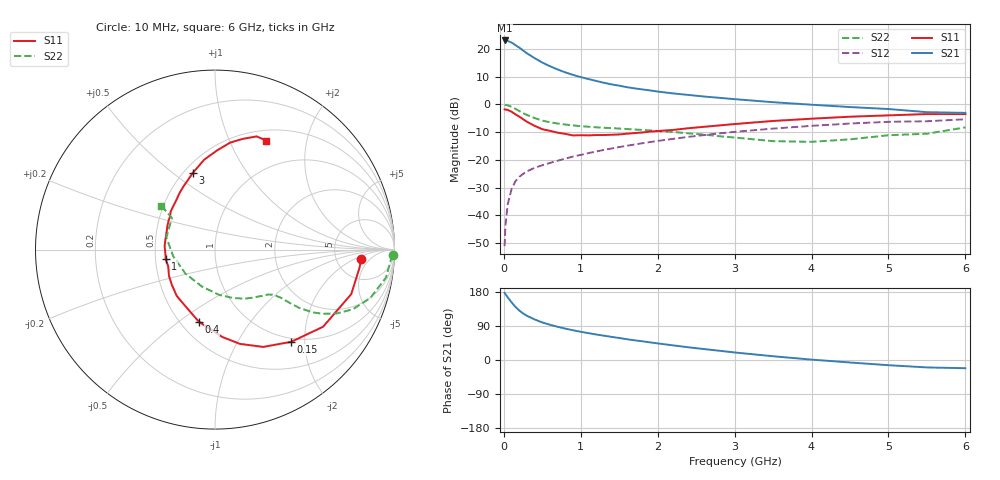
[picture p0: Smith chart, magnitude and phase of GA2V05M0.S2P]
! Infineon Technologies  Discrete & RF Semiconductors
! BF775
! Si NPN RF Bipolar Junction Transistor in SOT23
! VCE = 2 V  IC = 5 mA
! Common Emitter S-Parameters:  May  1996
# GHz  S  MA  R  50
!  f  S11  S21  S12  S22
! GHz  MAG  ANG  MAG  ANG  MAG  ANG  MAG  ANG
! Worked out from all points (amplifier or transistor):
!   36 points, 10 MHz to 6 GHz, reference 50 ohm
!   highest |S21| = 23.1 dB at 10 MHz (marker M1)
!   |S21| within 3 dB of that: start of sweep to 221 MHz
!   unconditionally stable (mu >= 1): 767.1 MHz to 3.983 GHz; 5.355 GHz to 5.765 GHz
!   at 250 MHz: K = 0.50, MSG = 22.2 dB, |S12| = -25.0 dB
!   at 1.4 GHz: K = 1.14, MAG = 9.2 dB, |S12| = -15.9 dB
!   at 6 GHz: K = 0.99, MSG = 1.2 dB, |S12| = -5.3 dB
!   lowest NFmin = 1.50 dB at 450 MHz
!   S11 on the Smith chart (normalised r, x): 10 MHz: 8.95, -2.91; 150 MHz: 0.93, -1.73; 400 MHz: 0.62, -0.60; 1 GHz: 0.57, -0.06; 3 GHz: 0.56, +0.59; 6 GHz: 0.63, +1.38
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0.01  0.8167 -3.8  14.24 177.2  0.0028 87.8  0.99 -1.8
0.02  0.8112 -7.3  14.04 173.9  0.0064 83.1  0.9798 -3.7
0.05  0.7986 -18.1  13.96 165.5  0.0158 79.7  0.966 -9.2
0.1  0.7399 -35.5  13.07 152.3  0.0296 71.6  0.9065 -17.3
0.15  0.6666 -50.4  11.74 140.3  0.0412 65.6  0.837 -23.4
0.2  0.6053 -63.6  10.61 130.7  0.0495 61.2  0.7639 -27.8
0.25  0.5433 -75.2  9.392 122.9  0.0561 57.9  0.6978 -30.8
0.3  0.4885 -85.2  8.358 116.7  0.0625 56.5  0.6474 -32.7
0.4  0.4118 -102.6  6.846 107.1  0.0721 54.1  0.5697 -34.7
0.5  0.3584 -116.6  5.691 99.0  0.0803 53.8  0.5129 -35.5
0.6  0.3347 -129.5  4.883 93.0  0.0885 54.1  0.4778 -35.9
0.8  0.2949 -150.4  3.781 82.8  0.1062 54.8  0.435 -36.8
1  0.2796 -169.2  3.113 74.5  0.1235 55.6  0.4072 -38.0
1.1  0.2774 -177.0  2.868 70.9  0.133 55.7  0.3972 -39.2
1.3  0.2815 169.2  2.463 64.2  0.1518 55.4  0.3807 -41.5
1.6  0.2977 152.7  2.05 54.8  0.1803 54.2  0.3608 -46.1
2.2  0.3481 128.6  1.582 38.6  0.2403 50.1  0.3203 -58.7
3  0.444 106.3  1.247 19.9  0.321 41.7  0.2538 -84.6
3.5  0.505 96.8  1.099 9.9  0.3676 35.5  0.2184 -109.4
4.5  0.6022 81.9  0.899 -6.6  0.4537 22.3  0.2355 -170.7
5.5  0.6719 69.8  0.727 -19.6  0.4988 7.7  0.2975 143.8
6  0.6714 64.7  0.706 -21.7  0.5409 3.6  0.3862 140.7
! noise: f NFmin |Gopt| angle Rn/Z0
0.45  1.5  0.28  29  0.34
0.9  1.8  0.25  59  0.34
